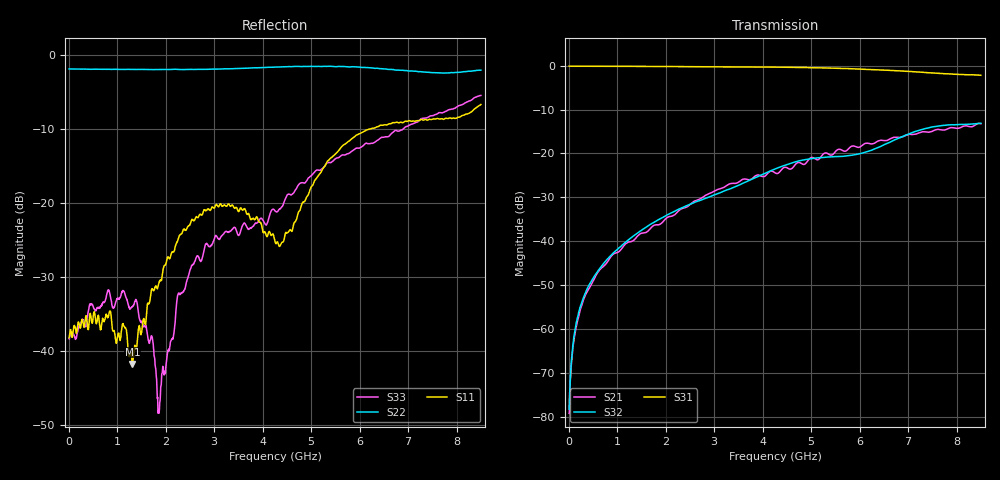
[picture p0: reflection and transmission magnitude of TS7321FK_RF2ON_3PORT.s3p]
!Created with skrf (http://scikit-rf.org).
# GHz S RI R 50.0
!freq ReS11 ImS11 ReS12 ImS12 ReS13 ImS13
! ReS21 ImS21 ReS22 ImS22 ReS23 ImS23
! ReS31 ImS31 ReS32 ImS32 ReS33 ImS33
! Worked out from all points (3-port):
!   1601 points, 10 MHz to 8.5 GHz, reference 50 ohm
!   strongest paths, dB at 10 MHz, 2.132 GHz, 4.255 GHz, 6.378 GHz, 8.5 GHz:
!     S31: -0.1, -0.2, -0.4, -1.0, -2.2
!     S32: -78.2, -33.4, -23.5, -18.7, -13.2
!     S21: -79.1, -34.3, -24.4, -17.2, -13.2
!   lowest |S11| = -41.7 dB at 1.315 GHz (marker M1), VSWR 1.02, Z = 50.8 + j0.0165 ohm
!   |S11| at or under -10 dB: start of sweep to 6.218 GHz
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0.01  0.0123 5.65e-05  7.11e-05 7.57e-05  0.9838 -0.00448
      0.000102 4.32e-05  -0.8042 0.00387  6.58e-05 9.53e-05
      0.9837 -0.00459  0.00011 5.55e-05  0.0119 0.0023
0.1214313  0.0146 0.00296  8.36e-05 0.000833  0.982 -0.0373
           7.82e-05 0.000838  -0.8016 0.0407  8.23e-05 0.000889
           0.9819 -0.0374  6.6e-05 0.000914  0.0124 0.0016
0.3230688  0.0126 0.00743  -2.65e-05 0.00228  0.9767 -0.0989
           -5.25e-05 0.00229  -0.7953 0.1076  3.67e-05 0.00241
           0.9769 -0.0989  4.32e-05 0.0024  0.0139 0.00712
1.315338  0.00821 0.000163  -0.000958 0.01  0.8991 -0.3871
          -0.000973 0.01  -0.6902 0.4019  0.000196 0.0112
          0.8988 -0.3872  0.000213 0.0113  0.0179 0.00888
1.723919  0.0169 -0.02  -0.00211 0.0146  0.8411 -0.4967
          -0.00214 0.0146  -0.6164 0.5039  0.0012 0.016
          0.8411 -0.4965  0.0012 0.016  0.00679 0.0105
1.867188  0.0165 -0.0245  -0.00179 0.0154  0.8173 -0.5337
          -0.00184 0.0154  -0.5876 0.5404  0.0017 0.0177
          0.8173 -0.5333  0.00175 0.0178  0.00238 0.00318
2.631288  0.0464 -0.0662  -0.00245 0.0292  0.6633 -0.7076
          -0.0025 0.0292  -0.4001 0.6914  0.00695 0.0273
          0.6636 -0.7073  0.00696 0.0274  -0.0318 0.029
4.255  0.0117 -0.0542  0.024 0.0553  0.2226 -0.933
       0.0239 0.0553  0.049 0.8263  0.0378 0.0548
       0.2228 -0.9322  0.0378 0.0547  -0.0392 0.0794
5.915856  -0.2745 -0.076  0.0815 0.0881  -0.2874 -0.8689
          0.0813 0.0881  0.4107 0.7218  0.0897 0.0369
          -0.2869 -0.8688  0.0898 0.0369  -0.0856 0.218
8.5  -0.3256 0.3285  0.2105 -0.0593  -0.7434 -0.2222
     0.21 -0.0587  0.7646 0.1961  0.1585 -0.1526
     -0.7426 -0.222  0.1582 -0.1529  0.3096 0.4334
